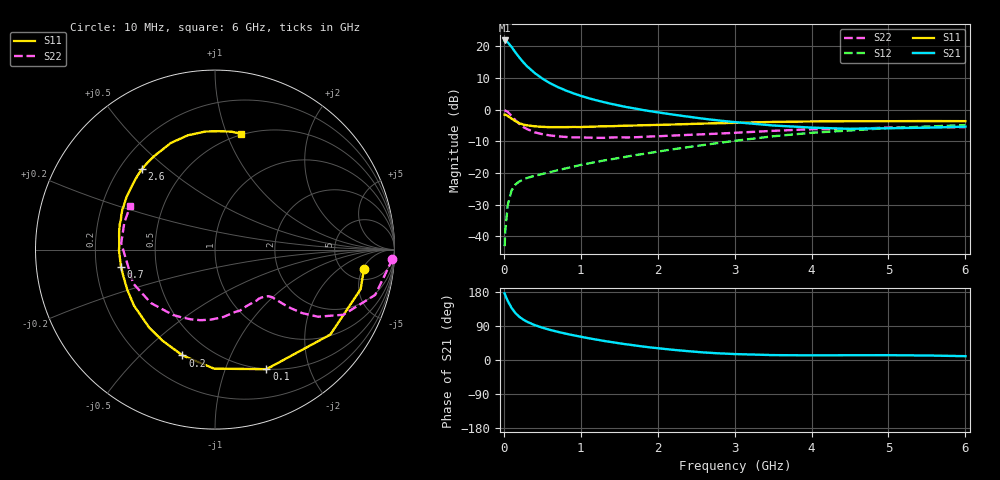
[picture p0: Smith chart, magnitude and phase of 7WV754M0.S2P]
! Infineon Technologies  Discrete & RF Semiconductors
! BFS17W
! Si NPN RF Bipolar Junction Transistor in SOT323
! VCE = 0.75 V  IC = 4 mA
! Common Emitter S-Parameters:  August  1999
# GHz  S  MA  R  50
!  f  S11  S21  S12  S22
! GHz  MAG  ANG  MAG  ANG  MAG  ANG  MAG  ANG
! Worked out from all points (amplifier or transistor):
!   36 points, 10 MHz to 6 GHz, reference 50 ohm
!   highest |S21| = 21.9 dB at 10 MHz (marker M1)
!   |S21| within 3 dB of that: start of sweep to 128.4 MHz
!   unconditionally stable (mu >= 1): 538.3 MHz to end of sweep
!   at 250 MHz: K = 0.56, MSG = 18.6 dB, |S12| = -22.1 dB
!   at 1.4 GHz: K = 1.38, MAG = 5.1 dB, |S12| = -15.6 dB
!   at 6 GHz: K = 1.13, MAG = -2.5 dB, |S12| = -4.8 dB
!   S11 on the Smith chart (normalised r, x): 10 MHz: 7.32, -5.34; 100 MHz: 0.50, -1.40; 200 MHz: 0.36, -0.68; 700 MHz: 0.31, -0.08; 2.6 GHz: 0.29, +0.41; 6 GHz: 0.49, +1.13
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0.01  0.8369 -7.5  12.46 175.8  0.007 85.4  0.9898 -2.9
0.02  0.8409 -15.2  12.45 170.2  0.0128 83.9  0.9675 -6.6
0.05  0.798 -36.4  11.67 156.2  0.0309 72.2  0.9274 -15.8
0.1  0.7253 -66.7  9.856 137.7  0.0531 57.4  0.8022 -26.9
0.15  0.6634 -90.4  8.103 123.9  0.0659 48.8  0.6849 -33.1
0.2  0.6167 -107.1  6.744 114.2  0.0736 44.8  0.6002 -36.1
0.25  0.5853 -120.1  5.687 107.0  0.0787 41.3  0.5369 -37.6
0.3  0.5685 -130.2  4.9 101.2  0.0836 40.6  0.4971 -38.4
0.4  0.5487 -145.4  3.819 92.2  0.0905 40.3  0.4403 -39.3
0.5  0.5375 -155.4  3.12 85.4  0.0967 41.0  0.4119 -39.9
0.6  0.5317 -163.3  2.632 79.5  0.1035 42.6  0.3933 -41.3
0.7  0.5322 -169.7  2.292 74.4  0.1109 44.3  0.3812 -43.3
0.9  0.5352 -179.6  1.824 65.5  0.1259 46.6  0.3667 -48.2
1.1  0.5393 172.1  1.526 57.5  0.142 48.7  0.363 -54.2
1.3  0.549 165.2  1.321 50.4  0.158 49.8  0.3607 -61.3
1.6  0.5622 156.6  1.102 41.2  0.1822 51.4  0.3652 -71.9
2.2  0.5855 141.5  0.84 26.9  0.2378 52.5  0.3917 -94.0
2.6  0.606 132.2  0.722 19.9  0.2781 51.7  0.4108 -108.8
3.5  0.6431 112.5  0.565 12.9  0.3812 45.9  0.4648 -140.2
4.5  0.66 94.7  0.5 12.6  0.471 34.7  0.4964 -172.2
5.5  0.6635 82.1  0.522 11.9  0.5438 24.3  0.5274 163.3
6  0.6613 77.2  0.542 10.1  0.5738 19.3  0.5308 152.6
